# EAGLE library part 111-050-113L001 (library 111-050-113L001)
NORCOMP - 111-050-113L001 - CONNECTOR, SCSI, PLUG, 50 POSITION, SOLDER Source: Datasheet
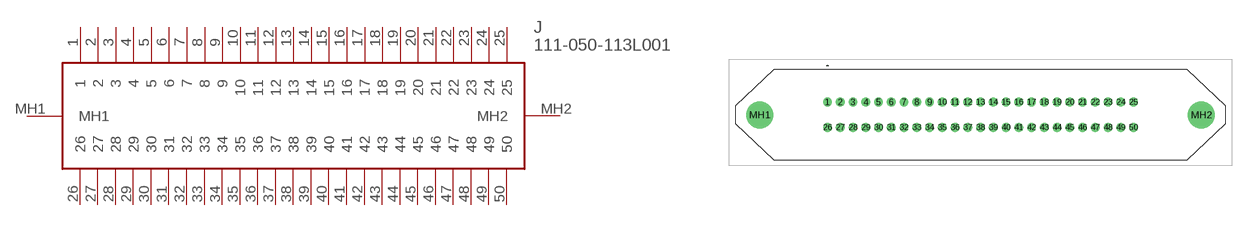
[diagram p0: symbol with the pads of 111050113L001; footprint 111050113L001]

Designator prefix J

## 111-050-113L001 (Description: NORCOMP - 111-050-113L001 - CONNECTOR, SCSI, PLUG, 50 POSITION, SOLDER; Height: 12.55mm; Manufacturer_Name: NorComp; Manufacturer_Part_Number: 111-050-113L001)  [111050113L001]
1  1
2  2
3  3
4  4
5  5
6  6
7  7
8  8
9  9
10  10
11  11
12  12
13  13
14  14
15  15
16  16
17  17
18  18
19  19
20  20
21  21
22  22
23  23
24  24
25  25
26  26
27  27
28  28
29  29
30  30
31  31
32  32
33  33
34  34
35  35
36  36
37  37
38  38
39  39
40  40
41  41
42  42
43  43
44  44
45  45
46  46
47  47
48  48
49  49
50  50
MH1  MH1
MH2  MH2

## Footprint 111050113L001 (pad centres in mm)
111-050-113L001-1
drill 1 pad 1.5: 1 0,0; 2 2.16,0; 3 4.32,0; 4 6.48,0; 5 8.64,0; 6 10.8,0; 7 12.96,0; 8 15.12,0; 9 17.28,0; 10 19.44,0; 11 21.6,0; 12 23.76,0; 13 25.92,0; 14 28.08,0; 15 30.24,0; 16 32.4,0; 17 34.56,0; 18 36.72,0; 19 38.88,0; 20 41.04,0; 21 43.2,0; 22 45.36,0; 23 47.52,0; 24 49.68,0; 25 51.84,0; 26 0,-4.29; 27 2.16,-4.29; 28 4.32,-4.29; 29 6.48,-4.29; 30 8.64,-4.29; 31 10.8,-4.29; 32 12.96,-4.29; 33 15.12,-4.29; 34 17.28,-4.29; 35 19.44,-4.29; 36 21.6,-4.29; 37 23.76,-4.29; 38 25.92,-4.29; 39 28.08,-4.29; 40 30.24,-4.29; 41 32.4,-4.29; 42 34.56,-4.29; 43 36.72,-4.29; 44 38.88,-4.29; 45 41.04,-4.29; 46 43.2,-4.29; 47 45.36,-4.29; 48 47.52,-4.29; 49 49.68,-4.29; 50 51.84,-4.29
drill 3.05 pad 4.575: MH1 -11.505,-2.145; MH2 63.345,-2.145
